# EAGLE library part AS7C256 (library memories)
RAM 32K x 8
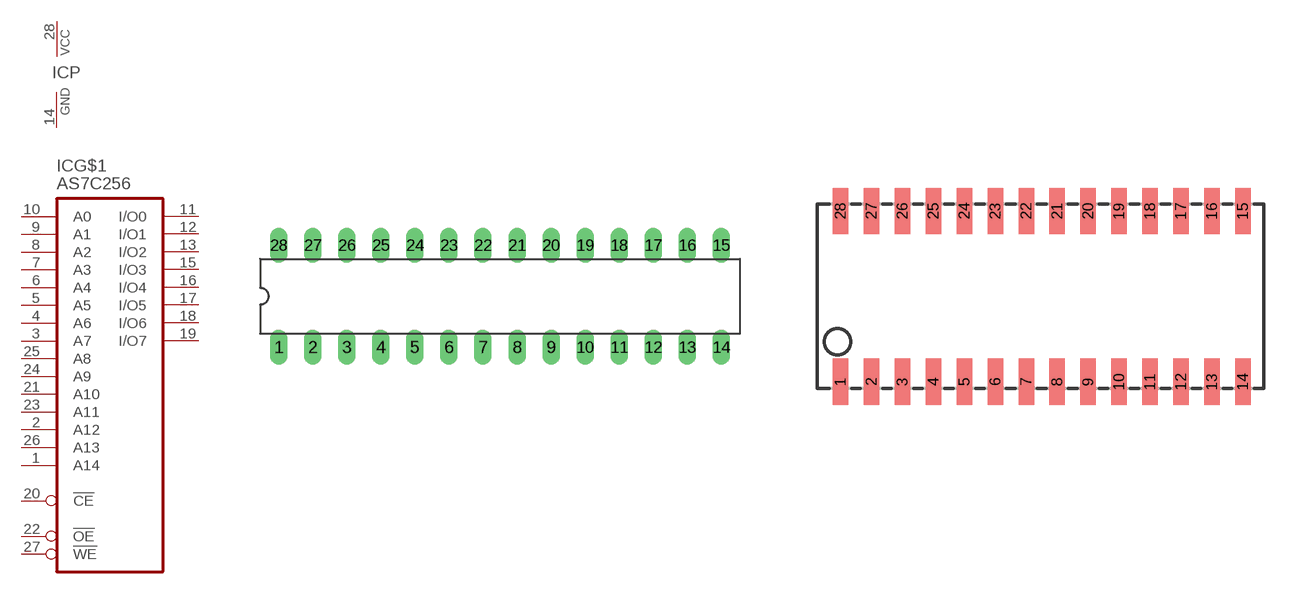
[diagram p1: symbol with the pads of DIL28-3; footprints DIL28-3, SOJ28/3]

Designator prefix IC; gates G$1=RAM32KX8 P=PWRN

## AS7C256P  [DIL28-3]
1  G$1:A14  in
2  G$1:A12  in
3  G$1:A7  in
4  G$1:A6  in
5  G$1:A5  in
6  G$1:A4  in
7  G$1:A3  in
8  G$1:A2  in
9  G$1:A1  in
10  G$1:A0  in
11  G$1:I/O0  hiz
12  G$1:I/O1  hiz
13  G$1:I/O2  hiz
14  P:GND  pwr
15  G$1:I/O3  hiz
16  G$1:I/O4  hiz
17  G$1:I/O5  hiz
18  G$1:I/O6  hiz
19  G$1:I/O7  hiz
20  G$1:!CE  in
21  G$1:A10  in
22  G$1:!OE  in
23  G$1:A11  in
24  G$1:A9  in
25  G$1:A8  in
26  G$1:A13  in
27  G$1:!WE  in
28  P:VCC  pwr

## AS7C256J  [SOJ28/3]
Pads as for DIL28-3

## AS7C256T  [TSOP28]
1  G$1:!OE  in
2  G$1:A11  in
3  G$1:A9  in
4  G$1:A8  in
5  G$1:A13  in
6  G$1:!WE  in
7  P:VCC  pwr
8  G$1:A14  in
9  G$1:A12  in
10  G$1:A7  in
11  G$1:A6  in
12  G$1:A5  in
13  G$1:A4  in
14  G$1:A3  in
15  G$1:A2  in
16  G$1:A1  in
17  G$1:A0  in
18  G$1:I/O0  hiz
19  G$1:I/O1  hiz
20  G$1:I/O2  hiz
21  P:GND  pwr
22  G$1:I/O3  hiz
23  G$1:I/O4  hiz
24  G$1:I/O5  hiz
25  G$1:I/O6  hiz
26  G$1:I/O7  hiz
27  G$1:!CE  in
28  G$1:A10  in

## Footprint DIL28-3 (pad centres in mm)
Dual In Line 0.3 inch
drill 0.813 long: 1 -16.51,-3.81; 2 -13.97,-3.81; 3 -11.43,-3.81; 4 -8.89,-3.81; 5 -6.35,-3.81; 6 -3.81,-3.81; 7 -1.27,-3.81; 8 1.27,-3.81; 9 3.81,-3.81; 10 6.35,-3.81; 11 8.89,-3.81; 12 11.43,-3.81; 13 13.97,-3.81; 14 16.51,-3.81; 15 16.51,3.81; 16 13.97,3.81; 17 11.43,3.81; 18 8.89,3.81; 19 6.35,3.81; 20 3.81,3.81; 21 1.27,3.81; 22 -1.27,3.81; 23 -3.81,3.81; 24 -6.35,3.81; 25 -8.89,3.81; 26 -11.43,3.81; 27 -13.97,3.81; 28 -16.51,3.81

## Footprint SOJ28/3 (pad centres in mm)
Small Outline J-Bend
smd 0.635 x 1.905: 1 -7.62,-3.505; 2 -6.35,-3.505; 3 -5.08,-3.505; 4 -3.81,-3.505; 5 -2.54,-3.505; 6 -1.27,-3.505; 7 0,-3.505; 8 1.27,-3.505; 9 2.54,-3.505; 10 3.81,-3.505; 11 5.08,-3.505; 12 6.35,-3.505; 13 7.62,-3.505; 14 8.89,-3.505; 15 8.89,3.505; 16 7.62,3.505; 17 6.35,3.505; 18 5.08,3.505; 19 3.81,3.505; 20 2.54,3.505; 21 1.27,3.505; 22 0,3.505; 23 -1.27,3.505; 24 -2.54,3.505; 25 -3.81,3.505; 26 -5.08,3.505; 27 -6.35,3.505; 28 -7.62,3.505

## Footprint TSOP28 (pad centres in mm)
smd 1.2 x 0.36: 1 -6.1,3.25; 2 -6.1,2.75; 3 -6.1,2.25; 4 -6.1,1.75; 5 -6.1,1.25; 6 -6.1,0.75; 7 -6.1,0.25; 8 -6.1,-0.25; 9 -6.1,-0.75; 10 -6.1,-1.25; 11 -6.1,-1.75; 12 -6.1,-2.25; 13 -6.1,-2.75; 14 -6.1,-3.25; 15 6.1,-3.25; 16 6.1,-2.75; 17 6.1,-2.25; 18 6.1,-1.75; 19 6.1,-1.25; 20 6.1,-0.75; 21 6.1,-0.25; 22 6.1,0.25; 23 6.1,0.75; 24 6.1,1.25; 25 6.1,1.75; 26 6.1,2.25; 27 6.1,2.75; 28 6.1,3.25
